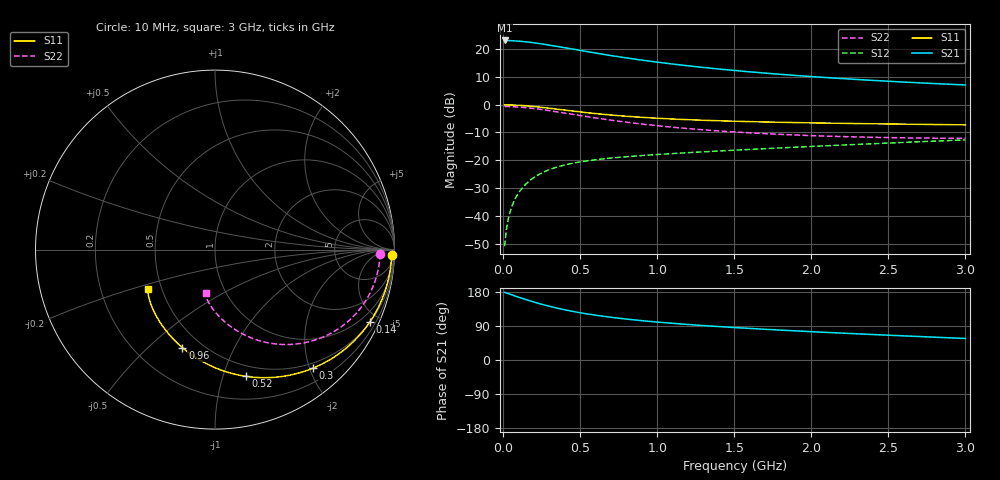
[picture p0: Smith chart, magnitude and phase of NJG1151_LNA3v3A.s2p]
! Created Fri Aug 03 14:35:09 2012
# hz S ma R 50
! 2 Port Network Data LNA section Port1:LNAIN  Port2:LNAOUT  VDD=3.3V,IDD=60mA  LNAIN connect GND Resistor(56kohm)
! freq  magS11  angS11  magS21  angS21  magS12  angS12  magS22  angS22
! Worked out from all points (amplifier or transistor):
!   300 points, 10 MHz to 3 GHz, reference 50 ohm
!   highest |S21| = 22.9 dB at 10 MHz (marker M1)
!   |S21| within 3 dB of that: start of sweep to 441.4 MHz
!   unconditionally stable (mu >= 1): nowhere
!   at 510 MHz: K = 0.30, MSG = 19.9 dB, |S12| = -20.4 dB
!   at 1.51 GHz: K = 0.69, MSG = 14.2 dB, |S12| = -16.3 dB
!   at 3 GHz: K = 0.89, MSG = 9.8 dB, |S12| = -12.7 dB
!   lowest NFmin = 0.19 dB at 10 MHz
!   S11 on the Smith chart (normalised r, x): 10 MHz: 25, -51; 140 MHz: 0.51, -4.43; 300 MHz: 0.41, -2.06; 520 MHz: 0.40, -1.19; 960 MHz: 0.39, -0.65; 3 GHz: 0.42, -0.23
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1e7  0.9847 -1.8  13.99 178.5  0.00292 62.9  0.9202 -1.4
3e7  0.9834 -5.5  13.95 175.7  0.00796 78.0  0.9188 -4.3
5e7  0.9807 -9.1  13.88 172.8  0.01314 79.9  0.9158 -7.1
9e7  0.9713 -16.3  13.68 167.3  0.02344 78.7  0.9052 -12.7
1.4e8  0.9521 -25.1  13.31 160.5  0.03581 75.1  0.8836 -19.6
1.8e8  0.9318 -31.9  12.93 155.4  0.04504 72.0  0.8608 -24.8
2.2e8  0.9085 -38.4  12.5 150.6  0.05355 68.9  0.8344 -29.8
2.6e8  0.8834 -44.5  12.04 146.0  0.0613 66.0  0.8058 -34.4
3e8  0.8574 -50.3  11.56 141.8  0.06829 63.4  0.776 -38.8
3.9e8  0.7997 -62.1  10.49 133.3  0.08154 58.3  0.7091 -47.5
5.1e8  0.7312 -75.5  9.178 124.0  0.09497 53.4  0.6275 -57.0
5.2e8  0.726 -76.4  9.078 123.3  0.09592 53.1  0.6212 -57.7
6.2e8  0.6795 -85.6  8.152 117.1  0.1044 50.4  0.5639 -64.1
7.2e8  0.6414 -93.5  7.362 111.7  0.1115 48.5  0.5155 -69.5
8.3e8  0.6074 -100.9  6.631 106.7  0.1182 47.1  0.4711 -74.5
9.6e8  0.5759 -108.3  5.918 101.6  0.1253 46.1  0.4285 -79.5
1.01e9  0.5658 -110.9  5.681 99.8  0.1279 45.8  0.4145 -81.2
1.23e9  0.5307 -120.3  4.821 92.8  0.1389 45.2  0.3648 -87.5
1.51e9  0.501 -129.2  4.04 85.4  0.1527 45.2  0.3217 -93.3
2.01e9  0.4687 -139.8  3.146 74.6  0.1781 45.5  0.2771 -99.5
2.51e9  0.4479 -146.1  2.597 65.2  0.2051 45.2  0.2555 -101.9
3e9  0.4324 -149.7  2.236 56.8  0.2326 44.1  0.2485 -101.5
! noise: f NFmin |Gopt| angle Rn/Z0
1e+07  0.189  0.7627  0.5413  0.161
3.4e+08  0.3941  0.5685  19.06  0.1615
6.7e+08  0.6927  0.3765  41.93  0.1601
1e+09  0.9994  0.2728  72.18  0.1574
1.33e+09  1.301  0.2485  104.4  0.154
1.67e+09  1.6  0.2696  129.6  0.1505
2e+09  1.878  0.3021  145.7  0.1478
2.33e+09  2.141  0.3329  157  0.1464
2.66e+09  2.389  0.3578  165.4  0.1473
3e+09  2.627  0.3764  172.3  0.1512
